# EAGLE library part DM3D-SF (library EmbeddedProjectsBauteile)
MicroSD Card
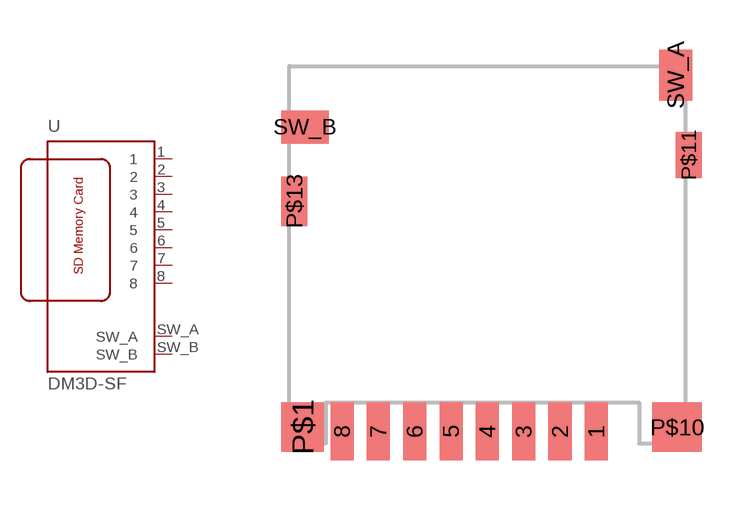
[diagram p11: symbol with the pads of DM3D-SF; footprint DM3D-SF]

Designator prefix -

## DM3D-SF (EP: 400106)  [DM3D-SF]
1  1  pas
2  2  pas
3  3  pas
4  4  pas
5  5  pas
6  6  pas
7  7  pas
8  8  pas
SW_A  SW_A  pas
SW_B  SW_B  pas

## Footprint DM3D-SF (pad centres in mm)
smd 0.7 x 1.75: 1 3.382,-5.701; 2 2.282,-5.701; 3 1.182,-5.701; 4 0.082,-5.701; 5 -1.018,-5.701; 6 -2.118,-5.701; 7 -3.218,-5.701; 8 -4.318,-5.701
smd 1.3 x 1.5: P$1 -5.518,-5.576
smd 1.5 x 1.5: P$10 5.832,-5.576
smd 0.8 x 1.4: P$11 6.182,2.674
smd 0.8 x 1.5: P$13 -5.768,1.274
smd 1 x 1.55: SW_A 5.782,5.099
smd 1.45 x 1: SW_B -5.443,3.524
